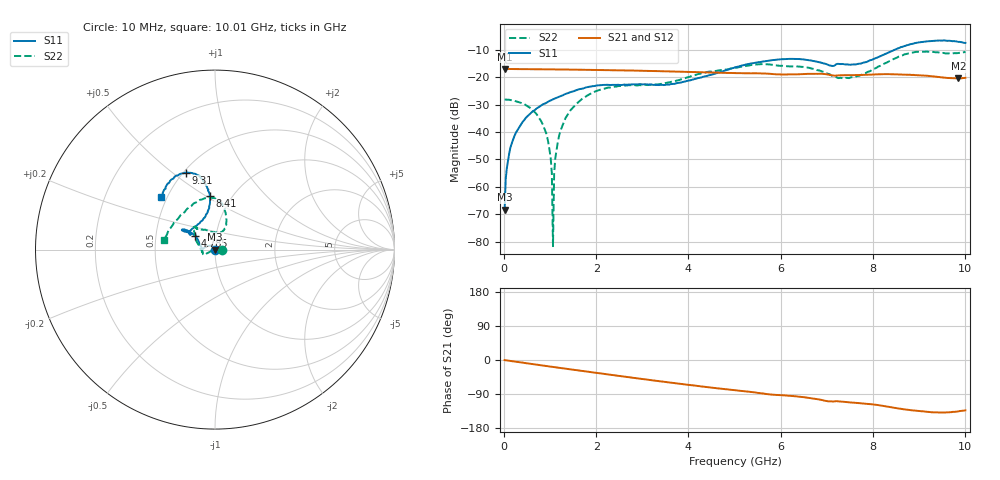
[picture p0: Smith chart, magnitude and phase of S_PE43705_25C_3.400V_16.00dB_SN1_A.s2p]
! Device ID: PE43705
! Serial: 1
! Insertion: A
! Impedance: 50 ohm
! Temp: 25C
! VDD: 3.400V
! Attenuation Step: 16.00dB
#  Hz  S  RI  R  50
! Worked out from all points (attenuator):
!   401 points, 10 MHz to 10.01 GHz, reference 50 ohm
!   highest |S21| = -17.03 dB at 10 MHz (marker M1); lowest = -20.5 dB at 9.86 GHz (marker M2)
!   lowest |S11| = -68.4 dB at 10 MHz (marker M3), VSWR 1.00, Z = 50 + j0.0382 ohm
!   |S11| at or under -10 dB: start of sweep to 8.48 GHz
!   |S22| runs from -81.6 to -10.7 dB; largest |S21 - S12| = 0.0018
!   S11 on the Smith chart (normalised r, x): 10 MHz: 1.00, +0.00; 4.785 GHz: 0.80, +0.12; 8.41 GHz: 0.79, +0.52; 9.31 GHz: 0.51, +0.56; 10.01 GHz: 0.46, +0.33
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1e7  1.95e-05 0.000382  0.1408 -0.000647  0.141 -0.000496  0.039 -7.13e-06
8.5e7  0.000215 0.00303  0.1403 -0.00386  0.1403 -0.00387  0.0387 0.000465
2.1e8  -0.000715 0.00785  0.1398 -0.00934  0.1398 -0.00929  0.0372 0.00251
7.85e8  -0.0193 0.0225  0.1351 -0.0328  0.1351 -0.0326  0.016 0.00469
9.35e8  -0.0263 0.0227  0.1329 -0.0388  0.133 -0.0387  0.00758 0.00257
9.85e8  -0.0291 0.0226  0.1323 -0.0407  0.1323 -0.0407  0.00447 0.0014
1.01e9  -0.0302 0.0223  0.1319 -0.0417  0.1319 -0.0416  0.00325 0.000807
1.06e9  -0.0326 0.0221  0.1309 -0.0434  0.131 -0.0434  5.17e-05 6.51e-05
1.11e9  -0.035 0.0212  0.1302 -0.0452  0.1303 -0.0452  -0.00299 -0.00147
1.16e9  -0.0374 0.021  0.1295 -0.0471  0.1295 -0.047  -0.00574 -0.00225
1.26e9  -0.0419 0.0193  0.1278 -0.0508  0.1279 -0.0507  -0.0118 -0.00461
1.685e9  -0.0608 0.00903  0.1192 -0.0654  0.1193 -0.0654  -0.0362 -0.0162
3.36e9  -0.0714 -0.00528  0.072 -0.1062  0.0721 -0.106  -0.0738 -0.00506
4.785e9  -0.1088 0.074  0.0273 -0.1164  0.0275 -0.1162  -0.1104 0.082
5.01e9  -0.1225 0.0873  0.021 -0.1165  0.0211 -0.1165  -0.1142 0.0937
6.685e9  -0.1704 0.1004  -0.0226 -0.1123  -0.0225 -0.1124  -0.0843 0.1146
7.435e9  -0.115 0.1252  -0.0391 -0.1014  -0.0389 -0.1015  0.0121 0.0961
8.36e9  -0.027 0.2848  -0.063 -0.0943  -0.0628 -0.0944  0.0621 0.1861
8.41e9  -0.0301 0.2966  -0.0645 -0.0923  -0.0644 -0.0929  0.0599 0.1952
9.31e9  -0.1632 0.4285  -0.0766 -0.0688  -0.0768 -0.0687  -0.0918 0.2722
9.86e9  -0.2755 0.3389  -0.0676 -0.0663  -0.0677 -0.0659  -0.246 0.122
1.001e10  -0.2987 0.2943  -0.0663 -0.0711  -0.0671 -0.0709  -0.2848 0.0546
